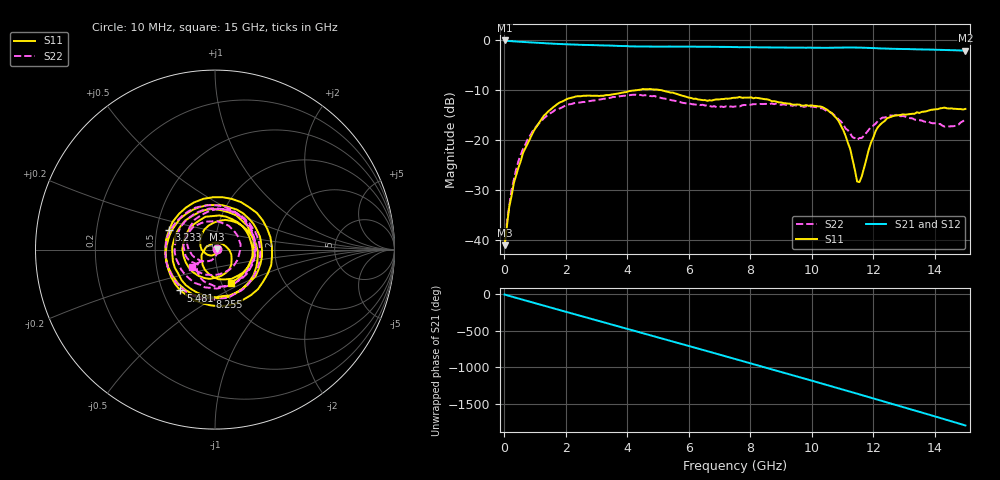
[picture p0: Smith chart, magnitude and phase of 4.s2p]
#  HZ  S  DB  R  50.00
! Rohde & Schwarz Vector Network Analyzer
! Rohde-Schwarz,ZNB3044-4Port,1351505044101548,4.21
! Created: UTC 8/5/2026, 7:44:10 PM
! freq[Hz]  db:S11  ang:S11  db:S21  ang:S21  db:S12  ang:S12  db:S22  ang:S22
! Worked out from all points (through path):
!   201 points, 10 MHz to 15 GHz, reference 50 ohm
!   highest |S21| = -0.07 dB at 10 MHz (marker M1); lowest = -2.1 dB at 15 GHz (marker M2)
!   group delay of S21, straight-line fit = 332 ps
!   lowest |S11| = -41.0 dB at 10 MHz (marker M3), VSWR 1.02, Z = 50.9 + j0.127 ohm
!   |S11| at or under -10 dB: start of sweep to 4.285 GHz; 5.112 GHz to end of sweep
!   |S22| runs from -41.1 to -10.9 dB; largest |S21 - S12| = 0.0054
!   S11 on the Smith chart (normalised r, x): 10 MHz: 1.02, +0.00; 3.233 GHz: 0.58, +0.14; 5.481 GHz: 0.62, -0.31; 8.255 GHz: 0.82, -0.46; 15 GHz: 1.11, -0.43
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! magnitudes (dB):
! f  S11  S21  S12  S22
! 10 MHz  -41.0  -0.1  -0.1  -41.1
! 159.9 MHz  -33.3  -0.2  -0.2  -33.1
! 234.8 MHz  -31.2  -0.2  -0.2  -30.0
! 459.7 MHz  -25.5  -0.3  -0.3  -24.2
! 759.5 MHz  -20.7  -0.4  -0.4  -19.8
! 1.434 GHz  -14.2  -0.7  -0.7  -14.8
! 2.558 GHz  -11.1  -1.0  -1.0  -12.4
! 3.233 GHz  -11.1  -1.1  -1.1  -11.7
! 5.032 GHz  -9.9  -1.3  -1.3  -11.4
! 5.481 GHz  -10.5  -1.3  -1.3  -12.1
! 6.606 GHz  -12.1  -1.3  -1.3  -13.0
! 7.505 GHz  -11.5  -1.4  -1.4  -13.2
! 8.255 GHz  -11.6  -1.5  -1.5  -12.8
! 10.05 GHz  -13.1  -1.5  -1.5  -13.3
! 10.88 GHz  -16.2  -1.5  -1.5  -15.9
! 11.25 GHz  -21.7  -1.5  -1.5  -18.6
! 11.48 GHz  -28.2  -1.5  -1.5  -19.9
! 11.55 GHz  -28.4  -1.5  -1.5  -19.6
! 12.08 GHz  -18.2  -1.6  -1.6  -16.7
! 12.53 GHz  -15.4  -1.7  -1.7  -15.0
! 14.33 GHz  -13.5  -2.0  -2.0  -17.3
! 15 GHz  -13.7  -2.1  -2.1  -15.8
